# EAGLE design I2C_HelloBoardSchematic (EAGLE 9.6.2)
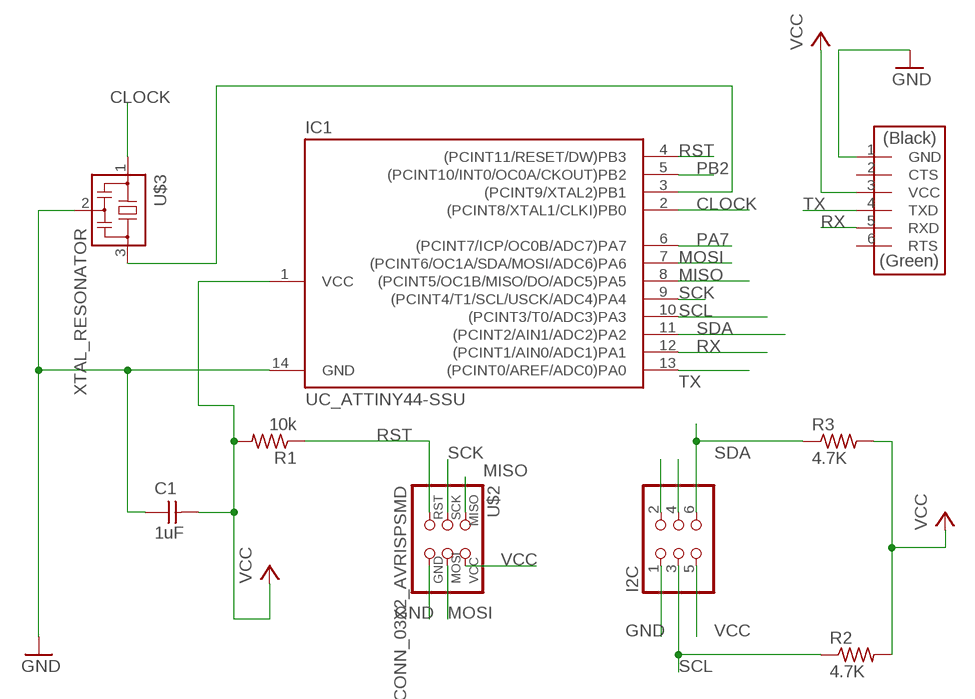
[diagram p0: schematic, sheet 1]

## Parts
C1  1uF  CAP_UNPOLARIZEDFAB  [C1206FAB]
I2C  CONN_03X2-PINHEAD-SMD  [2X03SMD]
IC1  UC_ATTINY44-SSU  [SOIC14]
R1  10k  R1206FAB  [R1206FAB]
R2  4.7K  R1206FAB  [R1206FAB]
R3  4.7K  R1206FAB  [R1206FAB]
U$1  CONN_06_FTDI-SMD-HEADER  [1X06SMD]
U$2  CONN_03X2_AVRISPSMD  [2X03SMD]
U$3  XTAL_RESONATOR  [EFOBM]

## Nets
CLOCK: IC1.2((PCINT8/XTAL1/CLKI)PB0) U$3.1
GND: C1.1 I2C.1 IC1.14(GND) U$1.1(GND) U$2.6(GND) U$3.2
MISO: IC1.8((PCINT5/OC1B/MISO/DO/ADC5)PA5) U$2.1(MISO)
MOSI: IC1.7((PCINT6/OC1A/SDA/MOSI/ADC6)PA6) U$2.4(MOSI)
N$2: IC1.3((PCINT9/XTAL2)PB1) U$3.3
N$6: I2C.4
N$7: I2C.2
PA7: IC1.6((PCINT7/ICP/OC0B/ADC7)PA7)
PB2: IC1.5((PCINT10/INT0/OC0A/CKOUT)PB2)
RST: IC1.4((PCINT11/RESET/DW)PB3) R1.1 U$2.5(RST)
RX: IC1.12((PCINT1/AIN0/ADC1)PA1) U$1.5(RXD)
SCK: IC1.9((PCINT4/T1/SCL/USCK/ADC4)PA4) U$2.3(SCK)
SCL: I2C.3 IC1.10((PCINT3/T0/ADC3)PA3) R2.1
SDA: I2C.6 IC1.11((PCINT2/AIN1/ADC2)PA2) R3.1
TX: IC1.13((PCINT0/AREF/ADC0)PA0) U$1.4(TXD)
VCC: C1.2 I2C.5 IC1.1(VCC) R1.2 R2.2 R3.2 U$1.3(VCC) U$2.2(VCC)
Unconnected: U$1.2(CTS) U$1.6(RTS)

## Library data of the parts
C1 = fab:CAP_UNPOLARIZED
I2C = fab:CONN_03X2-PINHEAD-SMD: PIN HEADER
IC1 = fab:UC_ATTINY44
R1-R3 = fab:R: Resistor (US Symbol)
U$1 = fab:CONN_06_FTDI-SMD-HEADER
U$2 = fab:CONN_03X2_AVRISP
U$3 = fab:XTAL_RESONATOR

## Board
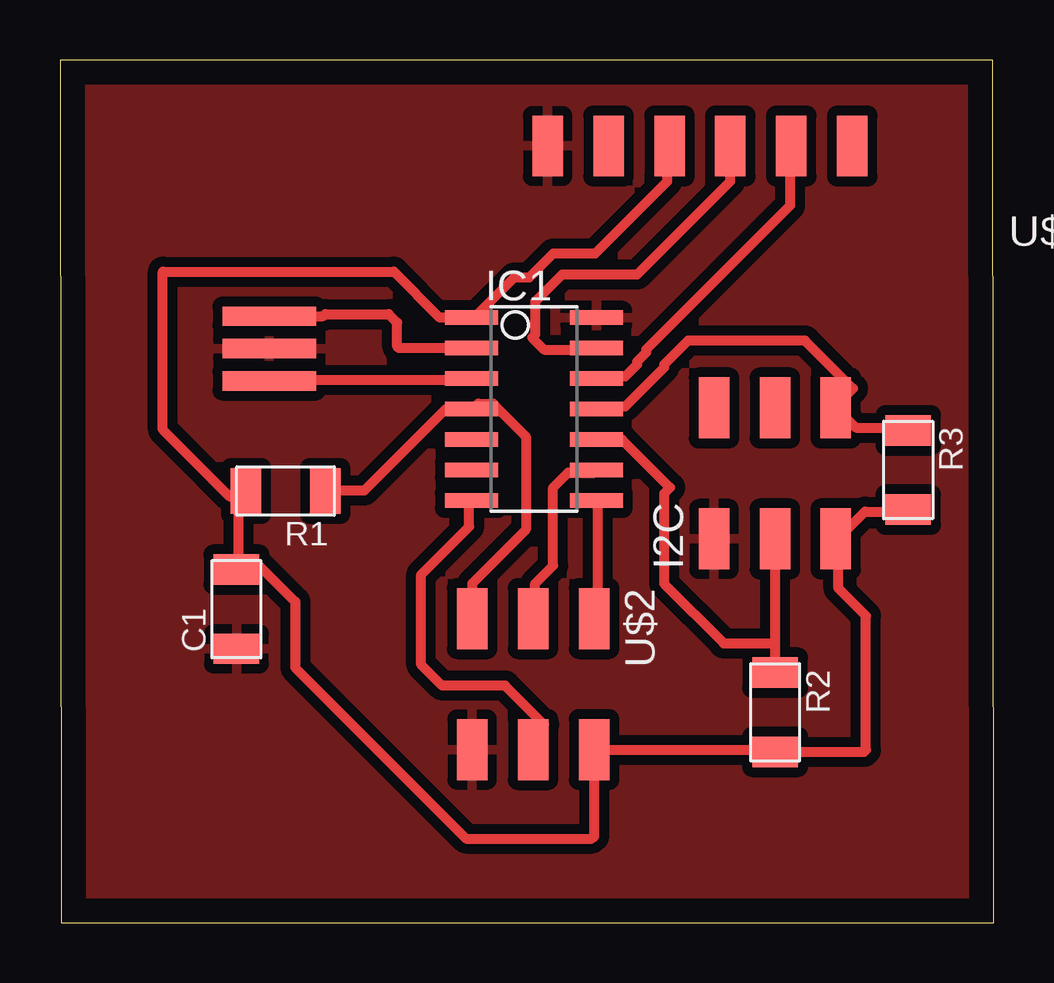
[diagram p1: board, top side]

Size 38.93 x 35.94 mm. Coordinates in mm from the lower left corner, seen from the top.
Outline: 0.05,0 38.93,0 38.88,35.94 0,35.94 0.05,0
Copper layers (1*16): Top 0.035mm / dielectric 1.5mm / Bottom 0.035mm
Design rules "default *": minimum track width 0.42mm, minimum drill 0.35mm, track to track 0.42mm, track to pad 0.42mm, pad to pad 0.42mm, via to via 4mm, smd to smd 0.4mm, copper to edge 40mil, drill to drill 6mil, minimum pad ring 10mil, minimum via ring 8mil, stop-mask expansion 4mil, vias tented up to drill 0mil, thermal gap 0.4mm

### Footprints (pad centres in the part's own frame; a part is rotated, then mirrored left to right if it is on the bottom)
C1206FAB = smd 1.27 x 1.905: 1 -1.651,0; 2 1.651,0
2X03SMD = smd 2.54 x 1.27: 1 -2.54,2.54; 2 2.92,2.54; 3 -2.54,0; 4 2.92,0; 5 -2.54,-2.54; 6 2.92,-2.54
SOIC14 = smd 0.61 x 2.21: 1 -3.81,-2.603; 2 -2.54,-2.603; 3 -1.27,-2.603; 4 0,-2.603; 5 1.27,-2.603; 6 2.54,-2.603; 7 3.81,-2.603; 8 3.81,2.603; 9 2.54,2.603; 10 1.27,2.603; 11 0,2.603; 12 -1.27,2.603; 13 -2.54,2.603; 14 -3.81,2.603
R1206FAB = smd 1.27 x 1.905: 1 -1.651,0; 2 1.651,0
1X06SMD = smd 2.54 x 1.27: 1 0,6.35; 2 0,3.81; 3 0,1.27; 4 0,-1.27; 5 0,-3.81; 6 0,-6.35
EFOBM = smd 0.8 x 3.9: 1 -1.35,0; 2 0,0; 3 1.35,0

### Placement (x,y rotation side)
C1  7.36,13.06 90 top
I2C  29.8,18.53 90 top
IC1  19.75,21.4 270 top
R1  9.4,17.98 180 top
R2  29.82,8.76 270 top
R3  35.36,18.86 270 top
U$1  26.68,32.36 90 top
U$2  19.73,10.13 270 top
U$3  8.72,23.92 270 top

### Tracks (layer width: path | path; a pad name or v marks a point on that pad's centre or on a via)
CLOCK
  Top 0.42: IC1.2 14.12,23.94 14.05,24 14.05,25 13.7,25.35 11.05,25.35 10.97,25.27 U$3.1
GND
  pour Top: -5.49,35.83 44.15,35.83 44.15,-12.54 -5.49,-12.54
MISO
  Top 0.42: IC1.8 22.43,17.5 22.43,12.88 22.3,12.75 U$2.1
MOSI
  Top 0.42: IC1.7 17.05,17.5 17.05,16.5 15.05,14.5 15.05,10.75 15.93,9.88 18.55,9.88 20.18,8.25 20.05,8.12 20.05,7.5 19.8,7.25 U$2.4
N$2
  Top 0.42: IC1.3 17.05,22.62 8.8,22.62 U$3.3
RST
  Top 0.42: R1.1 11.18,18 12.68,18 16.05,21.38 17.05,21.38 IC1.4 17.3,21.5 17.43,21.62 18.05,21.62 19.43,20.25 19.43,16.37 17.18,14.12 17.18,12.75 U$2.5
RX
  Top 0.42: IC1.12 22.43,22.75 23.55,22.75 24.05,23.25 24.05,23.38 24.43,23.75 24.43,23.88 30.43,29.88 30.43,32.25 U$1.5
SCK
  Top 0.42: IC1.9 22.3,18.75 21.18,18.75 20.55,18.12 20.55,14.88 19.8,14.12 19.8,12.75 U$2.3
SCL
  Top 0.42: IC1.10 22.43,20.12 23.43,20.12 25.43,18.12 25.18,17.88 25.18,14.12 27.67,11.64 29.8,11.64 | I2C.3 29.8,11.64 | 29.8,11.64 29.8,10.43 R2.1
SDA
  Top 0.42: R3.1 35.3,20.62 33.18,20.62 32.43,21.38 I2C.6 32.43,21.62 33.05,22.25 31.05,24.25 26.18,24.25 25.18,23.25 25.18,23.12 23.55,21.5 22.43,21.5 IC1.11
TX
  Top 0.42: IC1.13 22.3,23.88 20.18,23.88 19.68,24.38 19.8,24.5 19.8,25.88 20.93,27 24.05,27 27.93,30.88 27.93,32.25 U$1.4
VCC
  Top 0.42: R3.2 35.3,17.12 33.55,17.12 32.43,16 I2C.5 32.43,15.88 32.45,15.85 32.45,13.92 33.6,12.78 33.6,7.19 33.52,7.11 30.05,7.11 | U$1.3 25.3,32.25 25.3,30.88 22.3,27.88 20.55,27.88 19.55,26.88 18.93,26.88 17.3,25.25 17.18,25.25 IC1.1 15.83,25.21 13.91,27.13 13.91,27.12 4.29,27.12 4.29,20.54 7.08,17.75 7.3,17.75 R1.2 7.68,17.88 7.43,17.62 7.43,14.75 C1.2 7.55,14.62 8.05,15.12 9.8,13.38 9.8,10.62 16.93,3.5 22.17,3.5 22.27,3.6 U$2.2 29.96,7.21 30.05,7.11 | R2.2 30.05,7.11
